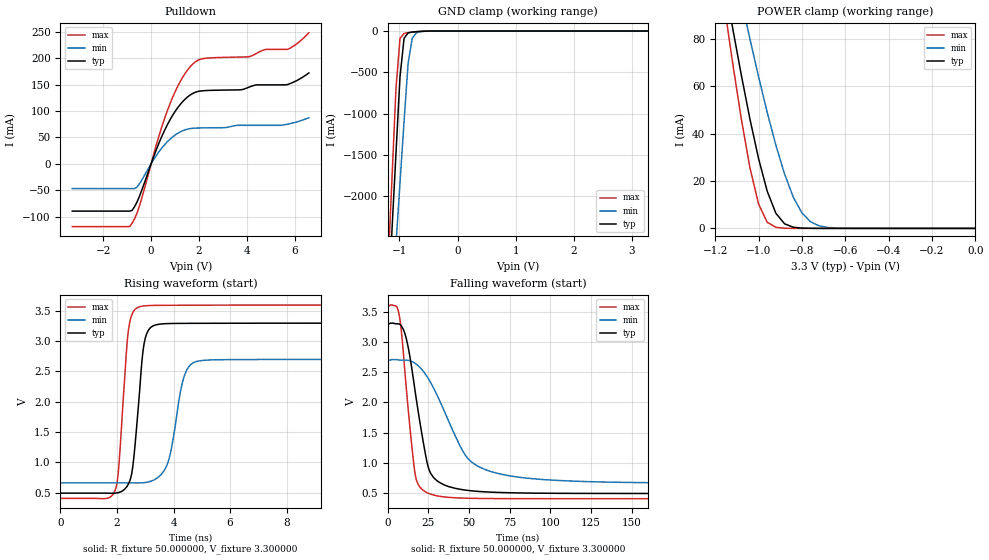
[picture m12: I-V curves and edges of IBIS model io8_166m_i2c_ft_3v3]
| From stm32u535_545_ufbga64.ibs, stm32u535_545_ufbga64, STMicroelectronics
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|   Model io8_166m_i2c_ft_3v3
[Model]  io8_166m_i2c_ft_3v3
Model_type I/O_open_drain
Polarity   Non-Inverting
Enable   Active-Low
Vinl =   0.990000V
Vinh =   2.310000V
Vmeas =  1.650000V
Cref =   50.000000pF
Rref =   100.000000M
Vref =   1.650000V
C_comp   3.523800pF   3.496000pF   3.564000pF
[Temperature Range]   25.000000   0.140000k   -40.000000
[Pullup Reference]   3.300000V   2.700000V   3.600000V
[Pulldown Reference]   0.0V   0.0V   0.0V
[POWER Clamp Reference]   3.300000V   2.700000V   3.600000V
[GND Clamp Reference]   0.0V   0.0V   0.0V
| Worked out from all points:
|   slope of the pulldown table from 0 to 0.495 V, typ, clamps not added: 8.73 ohm
|   GND clamp passes 1 mA (typ) near -0.50 V on its own axis
|   POWER clamp passes 1 mA (typ) near -0.85 V on its own axis
|   rising waveform, R_fixture 50.000000, V_fixture 3.300000: 20-80 % time 308ps typ, 455ps min, 272ps max; typ from 0.49 V to 3.3 V
|   falling waveform, R_fixture 50.000000, V_fixture 3.300000: 20-80 % time 10.1ns typ, 22.3ns min, 6.59ns max; typ from 3.3 V to 0.49 V
[Pulldown]
|Voltage   I(typ)   I(min)   I(max)
-3.3V     -89.72mA   -47.06mA   -119mA
-900mV    -89.72mA   -47.06mA   -119mA
-500mV    -62.92mA   -38.71mA   -81.44mA
300mV     36.2mA     21.01mA    48.7mA
800mV     84.07mA    46.96mA    114.8mA
1.3V      116.7mA    62.09mA    162.4mA
1.8V      134.4mA    67.39mA    191.2mA
2.3V      138.6mA    67.98mA    199.8mA
4.1V      145.2mA    72.79mA    202.7mA
4.8V      149.4mA    72.79mA    216.5mA
5.7V      149.8mA    74.8mA     216.5mA
6.6V      172mA      87.1mA     247.9mA
[GND_clamp]
|Voltage   I(typ)   I(min)   I(max)
-3.3V     -9.098A    -9.372A    -9.671A
-1.2V     -3.386A    -4.091A    -2.933A
-1.13V    -2.437A    -3.34A     -1.815A
-1.06V    -1.49A     -2.588A    -705.6mA
-990mV    -555.7mA   -1.839A    -89.03mA
-920mV    -88.12mA   -1.093A    -28.78mA
-850mV    -22.35mA   -387.4mA   -19.84mA
-780mV    -12.12mA   -88.01mA   -13.88mA
-710mV    -7.71mA    -22.52mA   -8.846mA
-640mV    -4.545mA   -7.864mA   -4.87mA
-360mV    -31.12uA   -173.5uA   -8.497uA
3.28V     0A         14.15nA    -7.901nA
[POWER_clamp]
|Voltage   I(typ)   I(min)   I(max)
-3.28V    1.355A     1.167A     1.664A
-1.16V    105.7mA    131.6mA    95.69mA
-1.12V    84.97mA    114mA      70.27mA
-1.08V    65.05mA    96.83mA    46.54mA
-1.04V    46.34mA    80.15mA    25.76mA
-1V       29.51mA    64.13mA    10.3mA
-960mV    15.69mA    48.99mA    2.571mA
-920mV    6.373mA    35.1mA     455.6uA
-840mV    490.7uA    13.24mA    11.36uA
-760mV    27.33uA    2.767mA    278.2nA
-640mV    347.6nA    134.1uA    16.76nA
0V        0A         19.95nA    0A
[Ramp]
| variable   typ   min   max
dV/dt_r  1.68607/0.50471n   1.22415/0.57522n   1.91789/0.30500n
dV/dt_f  1.68607/10.06522n   1.22415/22.25687n   1.91789/6.56642n
R_load = 50.000000
[Rising Waveform]
R_fixture= 50.000000
V_fixture= 3.300000
V_fixture_min= 2.700000
V_fixture_max= 3.600000
|time   V(typ)   V(min)   V(max)
0s        489.9mV    659.7mV    403.5mV
1.922ns   489.6mV    659.8mV    523.5mV
2.042ns   498.4mV    659.7mV    804.8mV
2.402ns   639.5mV    659.5mV    3.173V
2.803ns   2.186V     658.8mV    3.57V
3.163ns   3.214V     681.5mV    3.59V
3.764ns   3.291V     946.7mV    3.594V
4.364ns   3.295V     2.4V       3.595V
4.845ns   3.296V     2.669V     3.595V
19.94ns   3.3V       2.7V       3.6V
[Falling Waveform]
R_fixture= 50.000000
V_fixture= 3.300000
V_fixture_min= 2.700000
V_fixture_max= 3.600000
|time   V(typ)   V(min)   V(max)
0s        3.3V       2.7V       3.6V
6.406ns   3.3V       2.703V     3.521V
8.008ns   3.278V     2.7V       3.262V
11.21ns   3.074V     2.7V       2.288V
15.22ns   2.481V     2.671V     1.164V
17.62ns   2.038V     2.631V     709.8mV
26.43ns   821.6mV    2.325V     478.1mV
48.85ns   542.2mV    1.085V     411.1mV
74.47ns   502.5mV    784.9mV    404.5mV
398.8ns   489.9mV    659.7mV    403.5mV
